{attribute 'no_assign'}
FUNCTION_BLOCK FB_LN_IED_MUnn_UnnATVTR1 EXTENDS FB_AcsiCommonLogicalNodeClass
VAR_INPUT
	Beh: FB_DO_IED_MUnn_UnnATVTR1_Beh := (sClass:='ENS', bLinkResult:=THIS^.AddDataToContainer(ipData:=Beh));
	VolSv: FB_DO_IED_MUnn_UnnATVTR1_VolSv := (sClass:='SAV', bLinkResult:=THIS^.AddDataToContainer(ipData:=VolSv)); (*Voltage (sampled value)*)
END_VAR
VAR
END_VAR

END_FUNCTION_BLOCK
